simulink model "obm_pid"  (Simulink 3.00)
settings: Solver=ode5  StartTime=0.0  StopTime=20.0  FixedStep=Ts  RelTol=1e-3
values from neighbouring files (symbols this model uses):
  ac = 1-pc    [obm_sim_hinf.m]    (also in obm_sim_pid.m; obm_sim_smcrssi.m)
  coordinate_sw = 1    [obm_sim_hinf.m]    (also in obm_sim_pid.m; obm_sim_smcrssi.m)
  Ki1 = 2.9    [obm_sim_pid.m]
  Ki2 = 0.19    [obm_sim_pid.m]
  Kp1 = 2.3    [obm_sim_pid.m]
  Kp2 = 0.32    [obm_sim_pid.m]
  Kv1 = 0.05    [obm_sim_pid.m]
  Kv2 = 0.01    [obm_sim_pid.m]
  lim1 = 262.5e-3    (= 0.2625)    [obm_sim_hinf.m]    (also in obm_sim_pid.m; obm_sim_smcrssi.m = 1.3125)
  lim2 = 26.9e-3    (= 0.0269)    [obm_sim_hinf.m]    (also in obm_sim_pid.m; obm_sim_smcrssi.m = 0.1345)
  oscillation_start = 10    [obm_sim_hinf.m]    (also in obm_sim_pid.m; obm_sim_smcrssi.m)
  p = zeros(1,12)    [obm_pset.m]
  pc = input('Choice of the problem: enter 0 for attitude or 1 for postion.')    [obm_sim_hinf.m]    (also in obm_sim_pid.m = input('Selection of the problem: enter 0 for attitude or 1 f; obm_sim_smcrssi.m)
  r0 = 5    [obm_sim_hinf.m]    (also in obm_sim_pid.m; obm_sim_smcrssi.m)
  step1 = 30    [obm_sim_hinf.m]    (also in obm_sim_pid.m; obm_sim_smcrssi.m)
  step2 = 90    [obm_sim_hinf.m]    (also in obm_sim_pid.m; obm_sim_smcrssi.m)
  sw = input('choice of the ocsillation type: enter 1 for single; 2 for double; 3 for Bretschneider.')    [obm_hinf_syn.m]    (also in obm_sim_hinf.m = input('Choice of the ocsillation type: enter 1 for single; 2; obm_sim_pid.m = input('Selection of the ocsillation type: enter 1 for single; obm_sim_smcrssi.m = input('Choice of the ocsillation type: enter 1 for single; 2)
  Ts = 0.01    [obm_sim_hinf.m]    (also in obm_sim_pid.m; obm_sim_smcrssi.m = 0.001)
  X = 0.06    [obm_sim_hinf.m]    (also in obm_sim_pid.m; obm_sim_smcrssi.m)
  xy0 = obm_kinematics([r0;r0]*pi/180,0)    [obm_sim_hinf.m]    (also in obm_sim_pid.m; obm_sim_smcrssi.m)
  Y = 0.13    [obm_sim_hinf.m]    (also in obm_sim_pid.m; obm_sim_smcrssi.m)
undefined symbols (not defined in the file or in its folder): A1d, B1d, base_oscillation, C1d, D1d, obm_distH, obm_inv_kinematics, obm_kinematics, obm_sys
libraries: simulink3 x3

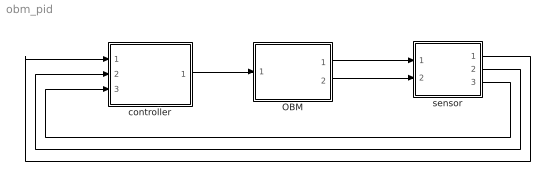
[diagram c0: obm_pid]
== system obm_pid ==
  OBM : Subsystem
  controller : Subsystem
  sensor : Subsystem
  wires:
  controller/1(control input) -> OBM/1(control input)
  OBM/1(q(t)) -> sensor/1(q(t))
  OBM/2(qb(t)) -> sensor/2(qb(t))
  sensor/1(qk) -> controller/1(qk)
  sensor/2(dqk) -> controller/2(dqk)
  sensor/3(qbk) -> controller/3(qbk)

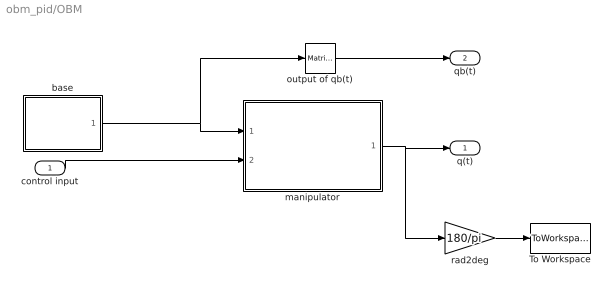
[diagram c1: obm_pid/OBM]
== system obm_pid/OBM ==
  control input : Inport  Port=1  PortWidth=-1  SampleTime=-1  DataType=auto
  To Workspace : ToWorkspace  VariableName=qout  SampleTime=-1  SaveFormat=Matrix
  base : Subsystem
  manipulator : Subsystem
  output of qb(t) : simulink3/Math/Matrix Gain  K=[1 0 0]
  rad2deg : Gain  Gain=180/pi  SaturateOnIntegerOverflow=on
  q(t) : Outport  Port=1
  qb(t) : Outport  Port=2
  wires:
  control input/1 -> manipulator/2(control input)
  base/1(oscillation) -> manipulator/1(base oscillation), output of qb(t)/1
  output of qb(t)/1 -> qb(t)/1
  rad2deg/1 -> To Workspace/1
  manipulator/1(q) -> q(t)/1, rad2deg/1

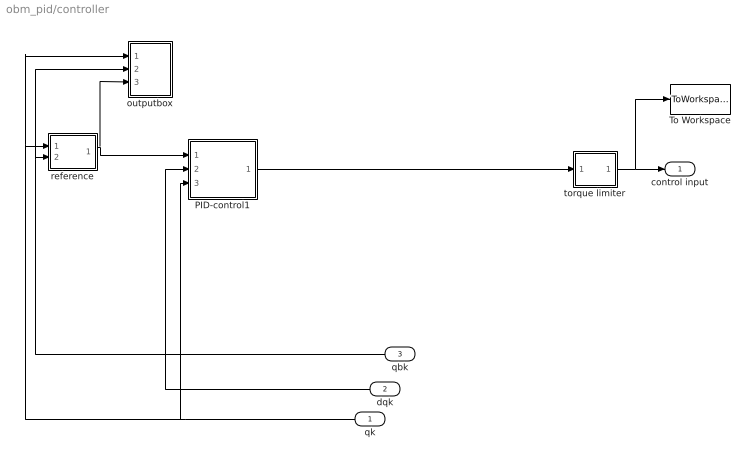
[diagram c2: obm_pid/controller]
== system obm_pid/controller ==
  qk : Inport  Orientation=left  Port=1  PortWidth=-1  SampleTime=-1  DataType=auto
  dqk : Inport  Orientation=left  Port=2  PortWidth=-1  SampleTime=-1  DataType=auto
  qbk : Inport  Orientation=left  Port=3  PortWidth=-1  SampleTime=-1  DataType=auto
  PID-control1 : Subsystem
  To Workspace : ToWorkspace  VariableName=torque  SampleTime=-1  SaveFormat=Matrix
  outputbox : Subsystem
  reference : Subsystem
  torque limiter : Subsystem
  control input : Outport  Port=1
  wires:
  torque limiter/1(Out) -> control input/1, To Workspace/1
  reference/1(r) -> outputbox/3(r), PID-control1/1(r)
  qbk/1 -> outputbox/2(qbk), reference/2(qbk)
  dqk/1 -> PID-control1/2(dqk)
  qk/1 -> outputbox/1(qk), reference/1(qk), PID-control1/3(qk)
  PID-control1/1(PD) -> torque limiter/1(In)

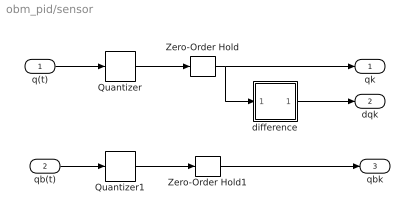
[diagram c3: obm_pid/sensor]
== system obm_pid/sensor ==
  q(t) : Inport  Port=1  PortWidth=-1  SampleTime=-1  DataType=auto
  qb(t) : Inport  Port=2  PortWidth=-1  SampleTime=-1  DataType=auto
  Quantizer : Quantizer  QuantizationInterval=rslv
  Quantizer1 : Quantizer  QuantizationInterval=rslv
  Zero-Order Hold : ZeroOrderHold  SampleTime=Ts
  Zero-Order Hold1 : ZeroOrderHold  SampleTime=Ts
  difference : Subsystem
  qk : Outport  Port=1
  dqk : Outport  Port=2
  qbk : Outport  Port=3
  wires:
  difference/1(Out1) -> dqk/1
  q(t)/1 -> Quantizer/1
  Quantizer/1 -> Zero-Order Hold/1
  Zero-Order Hold/1 -> qk/1, difference/1(In1)
  qb(t)/1 -> Quantizer1/1
  Quantizer1/1 -> Zero-Order Hold1/1
  Zero-Order Hold1/1 -> qbk/1

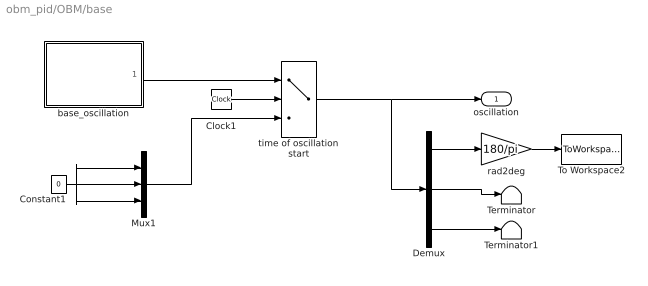
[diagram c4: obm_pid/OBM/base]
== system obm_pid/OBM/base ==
  Clock1 : Clock
  Constant1 : Constant  Value=0
  Demux : Demux  Outputs=3
  Mux1 : Mux  Inputs=3
  Terminator : Terminator
  Terminator1 : Terminator
  To Workspace2 : ToWorkspace  VariableName=qbout  SampleTime=-1  SaveFormat=Matrix
  base_oscillation : Subsystem
  rad2deg : Gain  Gain=180/pi  SaturateOnIntegerOverflow=on
  time of oscillation start : Switch  Threshold=oscillation_start
  oscillation : Outport  Port=1
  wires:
  Mux1/1 -> time of oscillation start/3
  Constant1/1 -> Mux1/2, Mux1/1, Mux1/3
  time of oscillation start/1 -> Demux/1, oscillation/1
  Demux/2 -> Terminator/1
  Demux/3 -> Terminator1/1
  Demux/1 -> rad2deg/1
  rad2deg/1 -> To Workspace2/1
  Clock1/1 -> time of oscillation start/2
  base_oscillation/1(base_oscilation) -> time of oscillation start/1

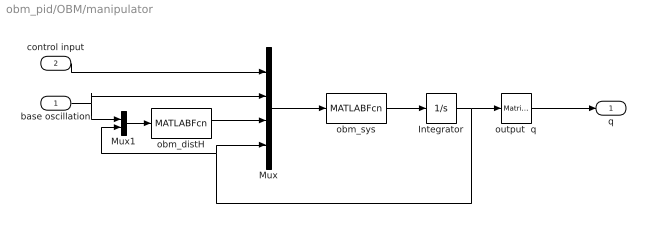
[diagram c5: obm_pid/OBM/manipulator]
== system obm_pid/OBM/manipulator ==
  base oscillation : Inport  Port=1  PortWidth=-1  SampleTime=-1  DataType=auto
  control input : Inport  Port=2  PortWidth=-1  SampleTime=-1  DataType=auto
  Integrator : Integrator  ExternalReset=none  InitialConditionSource=internal  InitialCondition=0  LimitOutput=off  UpperSaturationLimit=inf  LowerSaturationLimit=-inf  ShowSaturationPort=off  ShowStatePort=off  AbsoluteTolerance=auto
  Mux : Mux  Inputs=4
  Mux1 : Mux  Inputs=2
  obm_distH : MATLABFcn  MATLABFcn=obm_distH([u(4);u(5);u(6);u(7)],[u(1);u(2);u(3)],p)  OutputWidth=2  OutputSignalType=auto
  obm_sys : MATLABFcn  MATLABFcn=obm_sys([u(8);u(9);u(10);u(11)],[u(1);u(2)],u(3),[u(6);u(7)],p)  OutputWidth=4  OutputSignalType=auto
  output  q : simulink3/Math/Matrix Gain  K=[1 0 0 0; 0 1 0 0]
  q : Outport  Port=1
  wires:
  Mux1/1 -> obm_distH/1
  Mux/1 -> obm_sys/1
  obm_distH/1 -> Mux/3
  control input/1 -> Mux/1
  obm_sys/1 -> Integrator/1
  Integrator/1 -> output  q/1, Mux/4, Mux1/2
  base oscillation/1 -> Mux/2, Mux1/1
  output  q/1 -> q/1

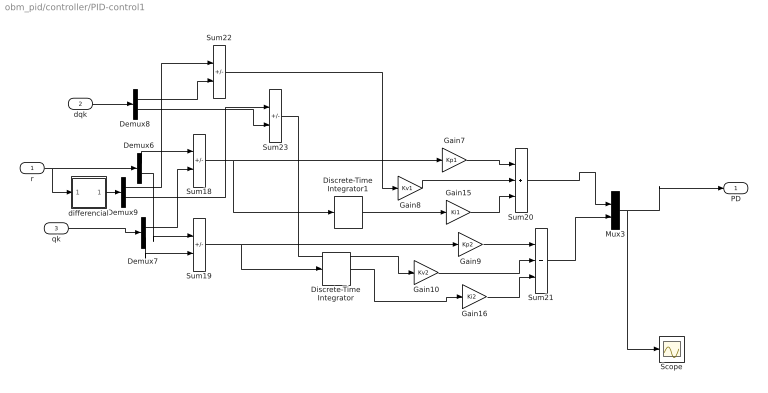
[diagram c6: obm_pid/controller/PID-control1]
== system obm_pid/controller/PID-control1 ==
  r : Inport  Port=1  PortWidth=-1  SampleTime=-1  DataType=auto
  dqk : Inport  Port=2  PortWidth=-1  SampleTime=-1  DataType=auto
  qk : Inport  Port=3  PortWidth=-1  SampleTime=-1  DataType=auto
  Demux{6..9} (4 alike) : Demux  Outputs=2
  Discrete-Time Integrator : DiscreteIntegrator  IntegratorMethod=BackwardEuler  ExternalReset=none  InitialConditionSource=internal  InitialCondition=0  LimitOutput=off  UpperSaturationLimit=inf  LowerSaturationLimit=-inf  ShowSaturationPort=off  ShowStatePort=off  SampleTime=0.01
  Discrete-Time Integrator1 : DiscreteIntegrator  IntegratorMethod=BackwardEuler  ExternalReset=none  InitialConditionSource=internal  InitialCondition=0  LimitOutput=off  UpperSaturationLimit=inf  LowerSaturationLimit=-inf  ShowSaturationPort=off  ShowStatePort=off  SampleTime=0.01
  Gain10 : Gain  Gain=Kv2  SaturateOnIntegerOverflow=on
  Gain15 : Gain  Gain=Ki1  SaturateOnIntegerOverflow=on
  Gain16 : Gain  Gain=Ki2  SaturateOnIntegerOverflow=on
  Gain7 : Gain  Gain=Kp1  SaturateOnIntegerOverflow=on
  Gain8 : Gain  Gain=Kv1  SaturateOnIntegerOverflow=on
  Gain9 : Gain  Gain=Kp2  SaturateOnIntegerOverflow=on
  Mux3 : Mux  Inputs=2
  Scope : Scope
  Sum{18..19,22..23} (4 alike) : Sum  Inputs=|+-  SaturateOnIntegerOverflow=on
  Sum20 : Sum  Inputs=|+++  SaturateOnIntegerOverflow=on
  Sum21 : Sum  Inputs=|+++  SaturateOnIntegerOverflow=on
  differencial : Subsystem
  PD : Outport  Port=1
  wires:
  Demux6/1 -> Sum18/1
  Demux7/1 -> Sum18/2
  Demux6/2 -> Sum19/1
  Demux7/2 -> Sum19/2
  Sum18/1 -> Gain7/1, Discrete-Time Integrator1/1
  Discrete-Time Integrator1/1 -> Gain15/1
  Gain7/1 -> Sum20/1
  Gain8/1 -> Sum20/2
  Gain15/1 -> Sum20/3
  Gain9/1 -> Sum21/1
  Gain10/1 -> Sum21/2
  Gain16/1 -> Sum21/3
  Sum19/1 -> Gain9/1, Discrete-Time Integrator/1
  Discrete-Time Integrator/1 -> Gain16/1
  Sum20/1 -> Mux3/1
  Sum21/1 -> Mux3/2
  qk/1 -> Demux7/1
  Mux3/1 -> PD/1, Scope/1
  dqk/1 -> Demux8/1
  r/1 -> Demux6/1, differencial/1(In1)
  differencial/1(Out1) -> Demux9/1
  Demux9/1 -> Sum22/1
  Demux8/1 -> Sum22/2
  Sum22/1 -> Gain8/1
  Demux8/2 -> Sum23/2
  Demux9/2 -> Sum23/1
  Sum23/1 -> Gain10/1

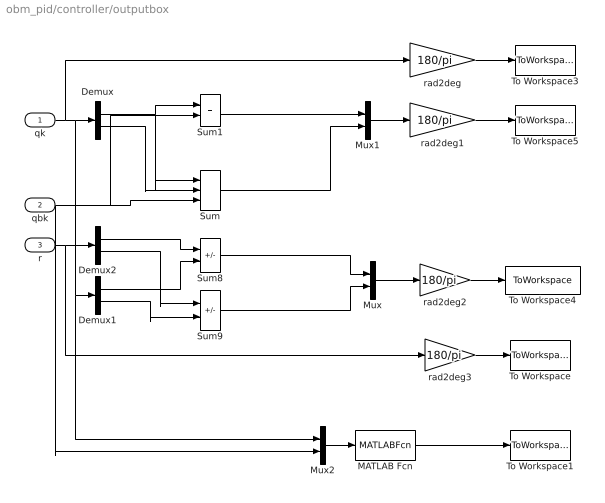
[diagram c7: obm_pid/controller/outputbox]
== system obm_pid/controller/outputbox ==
  qk : Inport  Port=1  PortWidth=-1  SampleTime=-1  DataType=auto
  qbk : Inport  Port=2  PortWidth=-1  SampleTime=-1  DataType=auto
  r : Inport  Port=3  PortWidth=-1  SampleTime=-1  DataType=auto
  Demux : Demux  Outputs=2
  Demux1 : Demux  Outputs=2
  Demux2 : Demux  Outputs=2
  MATLAB Fcn : MATLABFcn  MATLABFcn=norm(obm_kinematics([u(1);u(2)],u(3))-[X;Y])  OutputWidth=1  OutputSignalType=auto
  Mux : Mux  Inputs=2
  Mux1 : Mux  Inputs=2
  Mux2 : Mux  Inputs=2
  Sum : Sum  Inputs=|+++  SaturateOnIntegerOverflow=on
  Sum1 : Sum  Inputs=|++  SaturateOnIntegerOverflow=on
  Sum8 : Sum  Inputs=|+-  SaturateOnIntegerOverflow=on
  Sum9 : Sum  Inputs=|+-  SaturateOnIntegerOverflow=on
  To Workspace : ToWorkspace  VariableName=rqout  SampleTime=-1  SaveFormat=Matrix
  To Workspace1 : ToWorkspace  VariableName=xyout  SampleTime=-1  SaveFormat=Matrix
  To Workspace3 : ToWorkspace  VariableName=qkout  SampleTime=-1  SaveFormat=Matrix
  To Workspace4 : ToWorkspace  VariableName=qkerror_out  SampleTime=Ts  SaveFormat=Matrix
  To Workspace5 : ToWorkspace  VariableName=gqkout  SampleTime=-1  SaveFormat=Matrix
  rad2deg{,1..3} (4 alike) : Gain  Gain=180/pi  SaturateOnIntegerOverflow=on
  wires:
  qk/1 -> rad2deg/1, Demux/1, Demux1/1, Mux2/1
  Mux1/1 -> rad2deg1/1
  Demux/2 -> Sum/2
  Sum1/1 -> Mux1/1
  rad2deg1/1 -> To Workspace5/1
  rad2deg/1 -> To Workspace3/1
  Sum/1 -> Mux1/2
  Demux2/1 -> Sum8/1
  Demux2/2 -> Sum9/1
  Demux1/2 -> Sum9/2
  Sum8/1 -> Mux/1
  Sum9/1 -> Mux/2
  Mux/1 -> rad2deg2/1
  Demux1/1 -> Sum8/2
  rad2deg2/1 -> To Workspace4/1
  Demux/1 -> Sum1/1, Sum/1
  rad2deg3/1 -> To Workspace/1
  r/1 -> Demux2/1, rad2deg3/1
  Mux2/1 -> MATLAB Fcn/1
  qbk/1 -> Sum/3, Sum1/2, Mux2/2
  MATLAB Fcn/1 -> To Workspace1/1

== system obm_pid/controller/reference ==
  qk : Inport  Port=1  PortWidth=-1  SampleTime=-1  DataType=auto
  qbk : Inport  Port=2  PortWidth=-1  SampleTime=-1  DataType=auto
  Sum : Sum  Inputs=|++  SaturateOnIntegerOverflow=on
  ac switch : Gain  Gain=ac  SaturateOnIntegerOverflow=on
  attide control : Subsystem
  pc switch : Gain  Gain=pc  SaturateOnIntegerOverflow=on
  position control : Subsystem
  r : Outport  Port=1
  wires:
  qk/1 -> attide control/1(In1)
  qbk/1 -> attide control/2(In2), position control/1(qbk)
  attide control/1(Out1) -> ac switch/1
  position control/1(r2) -> pc switch/1
  ac switch/1 -> Sum/1
  pc switch/1 -> Sum/2
  Sum/1 -> r/1

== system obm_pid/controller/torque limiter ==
  In : Inport  Port=1  PortWidth=-1  SampleTime=-1  DataType=auto
  Demux1 : Demux  Outputs=2
  Mux1 : Mux  Inputs=2
  Saturation : Saturate  UpperLimit=lim1  LowerLimit=-lim1
  Saturation1 : Saturate  UpperLimit=lim2  LowerLimit=-lim2
  To Workspace1 : ToWorkspace  VariableName=torout2  SampleTime=-1  SaveFormat=Matrix
  Out : Outport  Port=1
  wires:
  Saturation/1 -> Mux1/1
  Demux1/1 -> Saturation/1
  Demux1/2 -> Saturation1/1
  Saturation1/1 -> Mux1/2
  In/1 -> Demux1/1
  Mux1/1 -> Out/1, To Workspace1/1

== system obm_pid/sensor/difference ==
  In1 : Inport  Port=1  PortWidth=-1  SampleTime=-1  DataType=auto
  Gain12 : Gain  Gain=1/Ts  SaturateOnIntegerOverflow=on
  Sum23 : Sum  Inputs=|-+  SaturateOnIntegerOverflow=on
  Unit Delay5 : UnitDelay  X0=0  SampleTime=Ts
  Out1 : Outport  Port=1
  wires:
  Gain12/1 -> Out1/1
  Unit Delay5/1 -> Sum23/1
  Sum23/1 -> Gain12/1
  In1/1 -> Unit Delay5/1, Sum23/2

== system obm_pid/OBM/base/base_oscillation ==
  Clock3 : Clock
  Derivative6 : Derivative
  Derivative7 : Derivative
  Mux4 : Mux  Inputs=3
  base_oscillation : MATLABFcn  MATLABFcn=base_oscillation(u,sw)  OutputWidth=-1  OutputSignalType=auto
  base_oscilation : Outport  Port=1
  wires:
  Clock3/1 -> base_oscillation/1
  Derivative6/1 -> Mux4/3
  Derivative7/1 -> Mux4/2, Derivative6/1
  base_oscillation/1 -> Mux4/1, Derivative7/1
  Mux4/1 -> base_oscilation/1

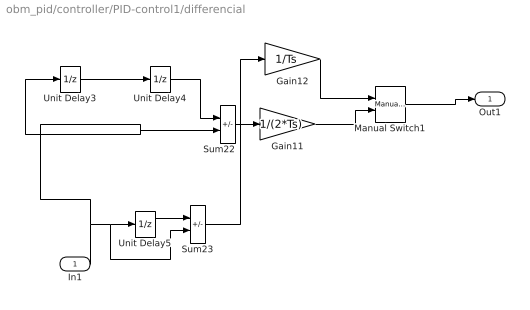
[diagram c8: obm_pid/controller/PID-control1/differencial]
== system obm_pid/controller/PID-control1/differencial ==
  In1 : Inport  Port=1  PortWidth=-1  SampleTime=-1  DataType=auto
  Gain11 : Gain  Gain=1/(2*Ts)  SaturateOnIntegerOverflow=on
  Gain12 : Gain  Gain=1/Ts  SaturateOnIntegerOverflow=on
  Manual Switch1 : simulink3/Nonlinear/Manual Switch  sw=1  action=0
  Sum22 : Sum  Inputs=|-+  SaturateOnIntegerOverflow=on
  Sum23 : Sum  Inputs=|-+  SaturateOnIntegerOverflow=on
  Unit Delay3 : UnitDelay  X0=0  SampleTime=Ts
  Unit Delay4 : UnitDelay  X0=0  SampleTime=Ts
  Unit Delay5 : UnitDelay  X0=0  SampleTime=Ts
  Out1 : Outport  Port=1
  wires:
  Sum22/1 -> Gain11/1
  Gain11/1 -> Manual Switch1/2
  In1/1 -> Sum22/2, Unit Delay3/1, Unit Delay5/1, Sum23/2
  Unit Delay3/1 -> Unit Delay4/1
  Unit Delay4/1 -> Sum22/1
  Unit Delay5/1 -> Sum23/1
  Sum23/1 -> Gain12/1
  Gain12/1 -> Manual Switch1/1
  Manual Switch1/1 -> Out1/1

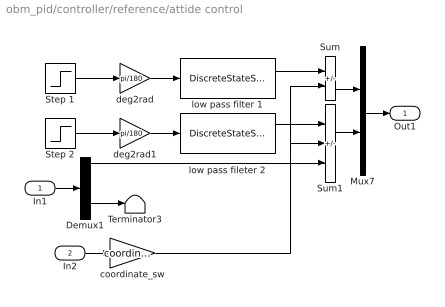
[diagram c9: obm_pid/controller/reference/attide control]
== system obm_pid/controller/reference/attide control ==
  In1 : Inport  Port=1  PortWidth=-1  SampleTime=-1  DataType=auto
  In2 : Inport  Port=2  PortWidth=-1  SampleTime=-1  DataType=auto
  Demux1 : Demux  Outputs=2
  Mux7 : Mux  Inputs=2
  Step 1 : Step  Time=10  Before=0  After=step1  SampleTime=Ts
  Step 2 : Step  Time=10  Before=0  After=step2  SampleTime=Ts
  Sum : Sum  Inputs=|+-  SaturateOnIntegerOverflow=on
  Sum1 : Sum  Inputs=|+--  SaturateOnIntegerOverflow=on
  Terminator3 : Terminator
  coordinate_sw : Gain  Gain=coordinate_sw  SaturateOnIntegerOverflow=on
  deg2rad : Gain  Gain=pi/180  SaturateOnIntegerOverflow=on
  deg2rad1 : Gain  Gain=pi/180  SaturateOnIntegerOverflow=on
  low pass fileter 2 : DiscreteStateSpace  A=A1d  B=B1d  C=C1d  D=D1d  X0=0  SampleTime=Ts
  low pass filter 1 : DiscreteStateSpace  A=A1d  B=B1d  C=C1d  D=D1d  X0=0  SampleTime=Ts
  Out1 : Outport  Port=1
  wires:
  Sum/1 -> Mux7/1
  Sum1/1 -> Mux7/2
  low pass filter 1/1 -> Sum/1
  low pass fileter 2/1 -> Sum1/1
  Demux1/2 -> Terminator3/1
  Demux1/1 -> Sum1/3
  coordinate_sw/1 -> Sum/2, Sum1/2
  deg2rad/1 -> low pass filter 1/1
  Step 1/1 -> deg2rad/1
  deg2rad1/1 -> low pass fileter 2/1
  Step 2/1 -> deg2rad1/1
  Mux7/1 -> Out1/1
  In1/1 -> Demux1/1
  In2/1 -> coordinate_sw/1

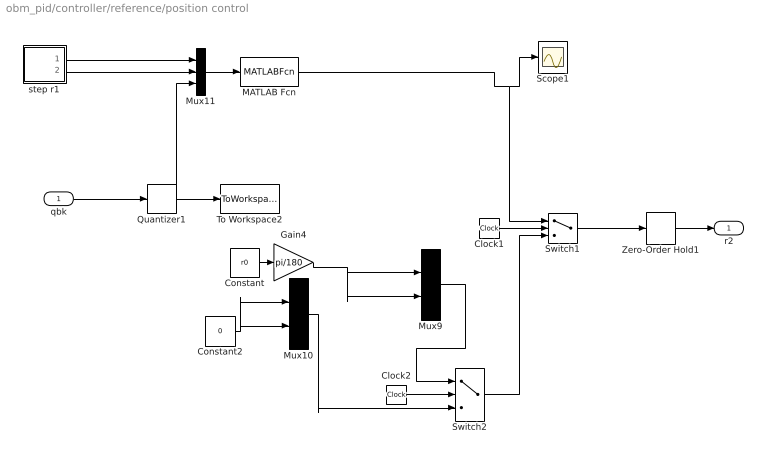
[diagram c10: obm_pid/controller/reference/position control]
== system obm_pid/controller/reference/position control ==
  qbk : Inport  Port=1  PortWidth=-1  SampleTime=-1  DataType=auto
  Clock1 : Clock
  Clock2 : Clock
  Constant : Constant  Value=r0
  Constant2 : Constant  Value=0
  Gain4 : Gain  Gain=pi/180  SaturateOnIntegerOverflow=on
  MATLAB Fcn : MATLABFcn  MATLABFcn=obm_inv_kinematics([u(1);u(2)],u(3))  OutputWidth=2  OutputSignalType=auto
  Mux10 : Mux  Inputs=2
  Mux11 : Mux  Inputs=3
  Mux9 : Mux  Inputs=2
  Quantizer1 : Quantizer  QuantizationInterval=rslv
  Scope1 : Scope
  Switch1 : Switch  Threshold=6
  Switch2 : Switch  Threshold=4
  To Workspace2 : ToWorkspace  VariableName=baseout2  SampleTime=-1  SaveFormat=Matrix
  Zero-Order Hold1 : ZeroOrderHold  SampleTime=Ts
  step r1 : Subsystem
  r2 : Outport  Port=1
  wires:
  Clock1/1 -> Switch1/2
  Clock2/1 -> Switch2/2
  Constant2/1 -> Mux10/2, Mux10/1
  Constant/1 -> Gain4/1
  Switch2/1 -> Switch1/3
  Mux9/1 -> Switch2/1
  Mux10/1 -> Switch2/3
  Gain4/1 -> Mux9/2, Mux9/1
  Zero-Order Hold1/1 -> r2/1
  Switch1/1 -> Zero-Order Hold1/1
  Quantizer1/1 -> To Workspace2/1, Mux11/3
  Mux11/1 -> MATLAB Fcn/1
  MATLAB Fcn/1 -> Scope1/1, Switch1/1
  step r1/1(x) -> Mux11/1
  step r1/2(y) -> Mux11/2
  qbk/1 -> Quantizer1/1

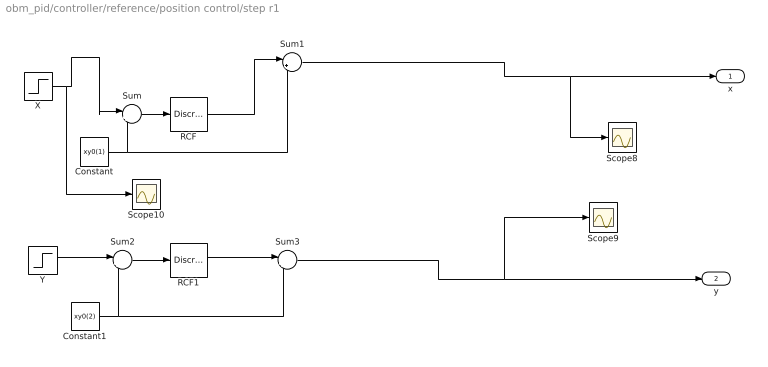
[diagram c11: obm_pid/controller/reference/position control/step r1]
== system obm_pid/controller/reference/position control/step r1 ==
  Constant : Constant  Value=xy0(1)
  Constant1 : Constant  Value=xy0(2)
  RCF : DiscreteStateSpace  A=A1d  B=B1d  C=C1d  D=D1d  X0=0  SampleTime=0.01
  RCF1 : DiscreteStateSpace  A=A1d  B=B1d  C=C1d  D=D1d  X0=0  SampleTime=0.01
  Scope10 : Scope
  Scope8 : Scope
  Scope9 : Scope
  Sum : Sum  Inputs=|+-  SaturateOnIntegerOverflow=on
  Sum1 : Sum  Inputs=|++  SaturateOnIntegerOverflow=on
  Sum2 : Sum  Inputs=|+-  SaturateOnIntegerOverflow=on
  Sum3 : Sum  Inputs=|++  SaturateOnIntegerOverflow=on
  X : Step  Time=6  Before=xy0(1)  After=X  SampleTime=0
  Y : Step  Time=6  Before=xy0(2)  After=Y  SampleTime=0
  x : Outport  Port=1
  y : Outport  Port=2
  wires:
  X/1 -> Scope10/1, Sum/1
  Sum1/1 -> x/1, Scope8/1
  Sum/1 -> RCF/1
  RCF/1 -> Sum1/1
  Constant/1 -> Sum/2, Sum1/2
  Y/1 -> Sum2/1
  Sum2/1 -> RCF1/1
  Constant1/1 -> Sum2/2, Sum3/2
  RCF1/1 -> Sum3/1
  Sum3/1 -> y/1, Scope9/1
